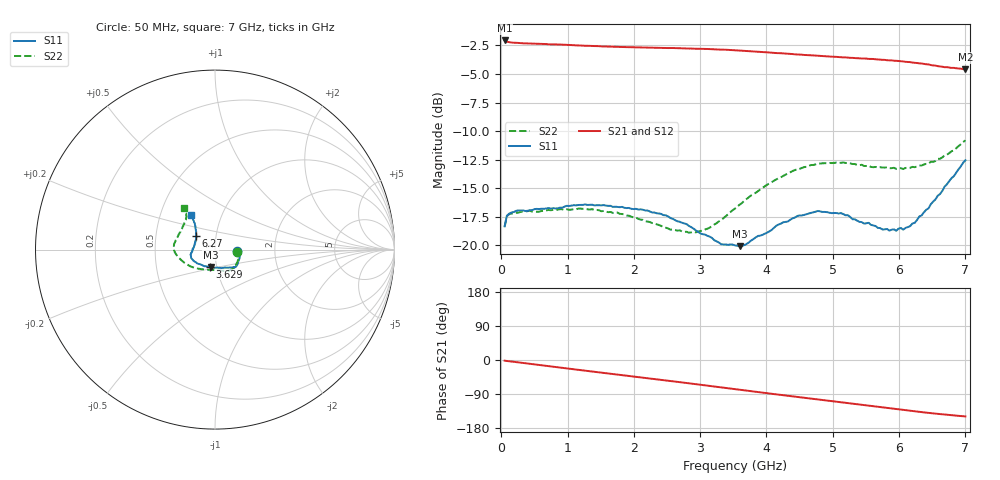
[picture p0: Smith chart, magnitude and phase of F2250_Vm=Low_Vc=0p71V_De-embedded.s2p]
! Integrated Device Technology
! Corporate Headquarters
! 6024 Silver Creek Valley Road
! San Jose, CA 95138  USA
! Phone:  1-408-284-8200
! Toll Free:  1-800-223-1366
! Webpage:  http://www.idt.com/
! Timing and RF Division
! 515 Groton Road, Suite 102
! Westford, MA 01886-6024
! Device:  F2250
! Description: Voltage Variable RF Attenuator
! Frequency:  50.0 -  6000.00 MHz
! Package:  3x3 mm Thin QFN Plastic Package: 16 pin
! Ports:  2 RF, 3 DC
!  Pin  1  = GND
!  Pin  2  = NC
!  Pin  3  = RF1  = Port 1
!  Pin  4  = NC
!  Pin  5  = GND
!  Pin  6  = GND
!  Pin  7  = GND
!  Pin  8  = GND
!  Pin  9  = NC
!  Pin 10  = RF2  = Port 2
!  Pin 11  = NC
!  Pin 12  = GND
!  Pin 13  = GND
!  Pin 14  = VCNTRL
!  Pin 15  = VDD
!  Pin 16  = VMODE
! Vcntrl:  0.710 Volts
! Vmode:  +0.000 Volts
! Vdd:  +3.30  Volts
! Current:  1.152 mA
! Data:  The device was measured on a the F2250 evaluation board which has
!  individual transmission lines to the RF pins.  Data was collected
!  using a calibrated network analyzer.  The evaluation board was
!  de-embedded using a TRL calibration technique.
!  The reference plane is the edge of the package pin.
! Misc:  SN 10
!  Action Tracker AT0258
! Date Measured:  2014-11-26
! Date:  2015-10-15  MJV
! Note:
!  Integrated Device Technology supplies this data as a sample of measured
!  data at the package pin for this product.  Your particular data for this
!  product may vary.
!  Data was taken at 25 degrees C.
!  Integrated Device Technology reserves the right to change this data at anytime.
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# GHz S dB R 50
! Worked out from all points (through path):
!   201 points, 50 MHz to 7 GHz, reference 50 ohm
!   highest |S21| = -2.06 dB at 50 MHz (marker M1); lowest = -4.6 dB at 7 GHz (marker M2)
!   group delay of S21, straight-line fit = 59.8 ps
!   lowest |S11| = -20.1 dB at 3.595 GHz (marker M3), VSWR 1.22, Z = 46.9 - j9.13 ohm
!   |S11| at or under -10 dB: start of sweep to end of sweep
!   |S22| runs from -18.9 to -10.8 dB; largest |S21 - S12| = 0.0014
!   S11 on the Smith chart (normalised r, x): 50 MHz: 1.27, -0.02; 3.629 GHz: 0.93, -0.18; 6.27 GHz: 0.80, +0.12; 7 GHz: 0.71, +0.29
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0.05  -18.34 -4.1  -2.06 -1.9  -2.06 -1.9  -18.38 -5.6
0.08475  -17.40 -4.3  -2.18 -2.5  -2.18 -2.5  -17.44 -5.4
0.22375  -16.98 -8.1  -2.27 -5.5  -2.27 -5.5  -17.15 -10.3
0.77975  -16.75 -24.5  -2.41 -17.7  -2.40 -17.7  -16.90 -31.7
1.2315  -16.46 -35.7  -2.52 -27.4  -2.52 -27.4  -16.81 -47.5
1.75275  -16.64 -42.4  -2.62 -38.4  -2.62 -38.4  -17.14 -59.2
2.37825  -17.22 -46.4  -2.72 -51.6  -2.72 -51.6  -18.22 -72.4
2.552  -17.62 -49.0  -2.72 -55.4  -2.72 -55.4  -18.63 -78.4
2.93425  -18.69 -59.5  -2.79 -63.8  -2.78 -63.8  -18.87 -97.6
3.3165  -19.91 -82.3  -2.87 -72.3  -2.86 -72.3  -17.79 -121.8
3.525  -20.01 -98.3  -2.91 -76.9  -2.92 -76.9  -16.78 -133.6
3.5945  -20.07 -103.5  -2.95 -78.5  -2.95 -78.5  -16.44 -136.9
3.62925  -20.07 -106.2  -2.96 -79.3  -2.96 -79.3  -16.30 -138.5
4.1505  -18.27 -139.2  -3.17 -90.7  -3.16 -90.7  -14.22 -161.4
4.7065  -17.11 -159.0  -3.38 -102.7  -3.38 -102.8  -12.97 -176.9
5.1235  -17.18 -169.0  -3.53 -111.6  -3.53 -111.6  -12.78 173.6
5.471  -18.10 -179.3  -3.64 -119.0  -3.64 -119.0  -13.05 165.8
5.85325  -18.71 166.2  -3.80 -127.1  -3.80 -127.1  -13.26 156.0
6.06175  -18.63 156.0  -3.90 -131.5  -3.91 -131.5  -13.33 149.7
6.27025  -17.79 144.3  -4.04 -136.0  -4.04 -136.0  -13.10 143.0
6.61775  -15.51 130.1  -4.34 -142.7  -4.34 -142.7  -12.42 131.6
7  -12.55 124.9  -4.58 -148.9  -4.59 -148.9  -10.81 127.1
